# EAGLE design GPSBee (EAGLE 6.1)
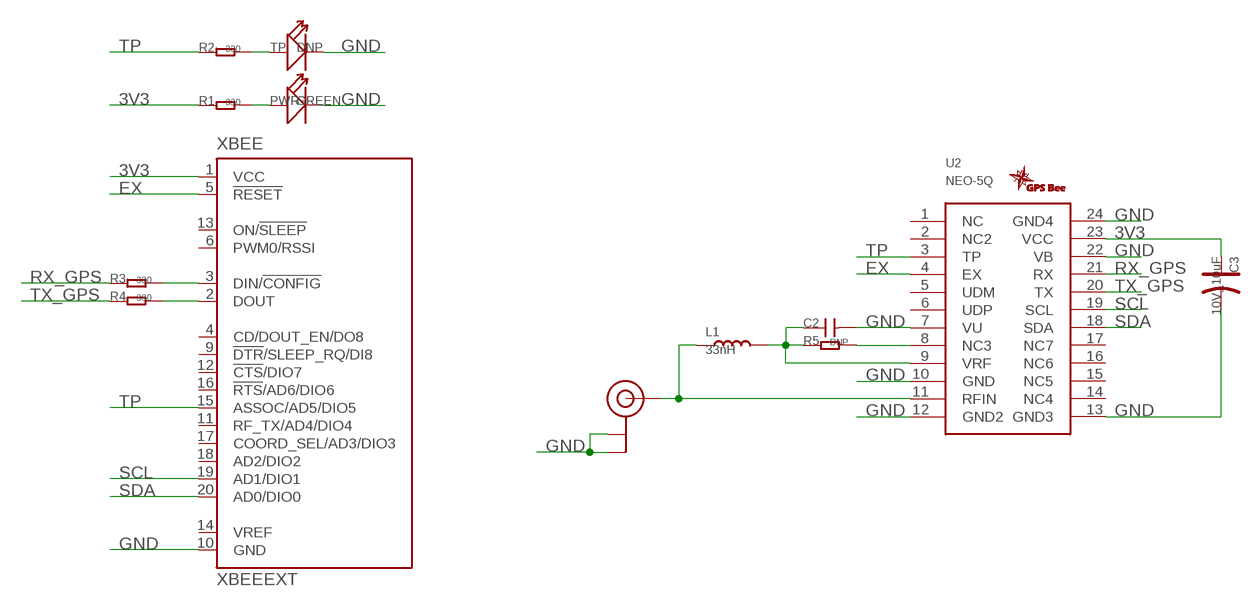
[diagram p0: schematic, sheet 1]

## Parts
C2  C-0603  [0603]
C3  10V_10uF  CAP-AVX-A  [AVX-A]
L1  33nH  L0603  [0603]
LOGO1  GPSLOGO_SLIK  [GPSLOGO]
PWR  GREEN  LED'0603'  [LED-0603]
R1  330  R-0603  [0603]
R2  330  R-0603  [0603]
R3  330  R-0603  [0603]
R4  330  R-0603  [0603]
R5  DNP  R-0603  [0603]
TP  DNP  LED'0603'  [LED-0603]
U2  NEO-5Q  [NEO-5Q]
U3  U.FL  [U.FL]
XBEE  XBEEEXT  [XBEE_PLUG]

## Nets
3V3: C3.+ R1.1 U2.23(VCC) XBEE.1(VCC)
EX: U2.4(EX) XBEE.5(!RESET)
GND: C2.2 C3.- PWR.- TP.- U2.7(VU) U2.10(GND) U2.12(GND2) U2.13(GND3) U2.22(VB) U2.24(GND4) U3.P$1(GND) U3.P$2(GND) XBEE.10(GND)
N$1: PWR.+ R1.2
N$2: L1.1 U2.11(RFIN) U3.P$3(SIGNAL)
N$3: C2.1 L1.2 R5.1 U2.9(VRF)
N$4: R3.2 XBEE.3(DIN/!CONFIG)
N$5: R2.2 TP.+
N$6: R4.2 XBEE.2(DOUT)
N$7: R5.2 U2.8(NC3)
RX_GPS: R3.1 U2.21(RX)
SCL: U2.19(SCL) XBEE.19(AD1/DIO1)
SDA: U2.18(SDA) XBEE.20(AD0/DIO0)
TP: R2.1 U2.3(TP) XBEE.15(ASSOC/AD5/DIO5)
TX_GPS: R4.1 U2.20(TX)
Unconnected: U2.1(NC) U2.2(NC2) U2.5(UDM) U2.6(UDP) U2.14(NC4) U2.15(NC5) U2.16(NC6) U2.17(NC7) XBEE.4(CD/DOUT_EN/DO8) XBEE.6(PWM0/RSSI) XBEE.9(!DTR!/SLEEP_RQ/DI8) XBEE.11(RF_TX/AD4/DIO4) XBEE.12(!CTS!/DIO7) XBEE.13(ON/!SLEEP) XBEE.14(VREF) XBEE.16(!RTS!/AD6/DIO6) XBEE.17(COORD_SEL/AD3/DIO3) XBEE.18(AD2/DIO2)

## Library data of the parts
C2 = Discrete:C*: Ceramic Capacitors
C3 = Discrete:CAP*: Electrolytic Capacitors,Tantalum Capacitors and Super Capacitors
L1 = Discrete:L*
LOGO1 = logo:GPSLOGO_SLIK
PWR TP = Discrete:LED*
R1-R5 = Discrete:R*
U2 = Seeed:NEO-5Q
U3 = SparkFun2:U.FL
XBEE = EXT_moudle:XBEE: XBee (TM) /XBee-PRO(TM) OEM RF Modules Source: MaxStream, Inc. xbee_productmanual.pdf

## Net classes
0 default: width 0.003 mm, drill 0.254 mm, clearance 0.152 mm

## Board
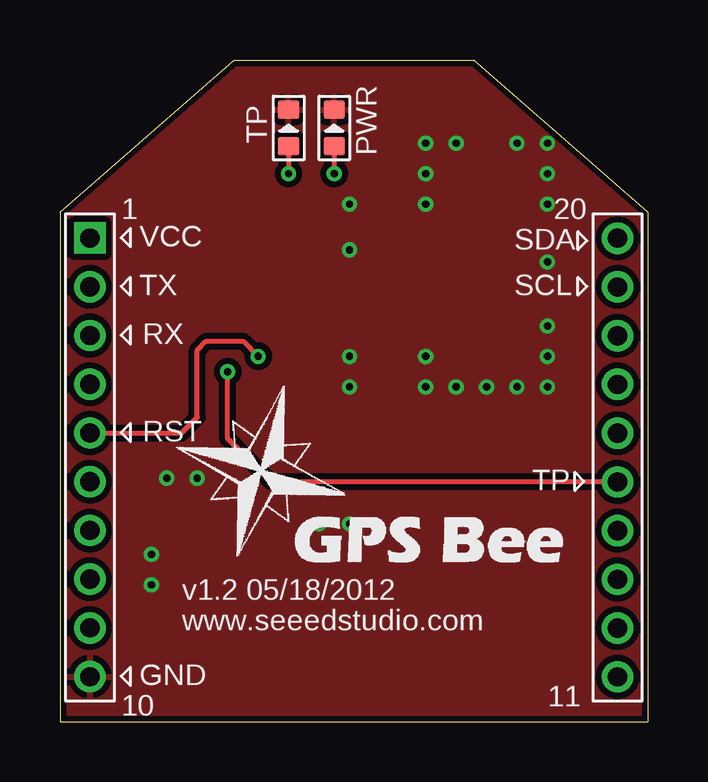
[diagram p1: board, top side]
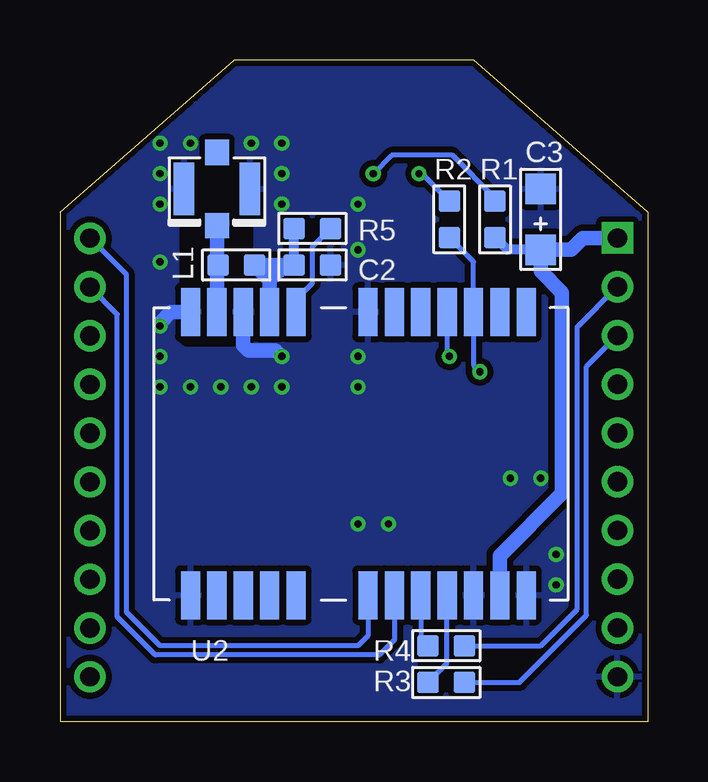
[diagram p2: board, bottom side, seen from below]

Size 24.5 x 27.6 mm. Coordinates in mm from the lower left corner, seen from the top.
Outline: 7.25,27.6 17.25,27.6 24.5,21.25 24.5,0 0,0 0,21.25 7.25,27.6
Copper layers (1*16): Top 0.035mm / dielectric 1.5mm / Bottom 0.035mm
Design rules: minimum track width 6mil, minimum drill 12mil, track to track 6mil, track to pad 6mil, pad to pad 6mil, via to via 6mil, smd to smd 0mil, copper to edge 10mil, drill to drill 10mil, minimum pad ring 10mil, minimum via ring 6mil, stop-mask expansion 2mil, vias tented up to drill 100mil, thermal gap 10mil
bRestrict: 4 lines

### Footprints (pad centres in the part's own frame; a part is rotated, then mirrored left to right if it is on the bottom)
0603 = smd 0.889 x 0.889: 1 -0.762,0; 2 0.762,0
AVX-A = smd 1.27 x 1.27: + -1.27,0; - 1.27,0
LED-0603 = smd 0.762 x 0.889: + -0.762,0; - 0.762,0
NEO-5Q = smd 2 x 0.8: 1 12,-14; 2 12,-12.9; 3 12,-11.8; 4 12,-10.7; 5 12,-9.6; 6 12,-8.5; 7 12,-7.4; 8 12,-4.4; 9 12,-3.3; 10 12,-2.2; 11 12,-1.1; 12 12,0; 13 0.2,0; 14 0.2,-1.1; 15 0.2,-2.2; 16 0.2,-3.3; 17 0.2,-4.4; 18 0.2,-7.4; 19 0.2,-8.5; 20 0.2,-9.6; 21 0.2,-10.7; 22 0.2,-11.8; 23 0.2,-12.9; 24 0.2,-14
U.FL = smd 2.2 x 0.85: P$1 0,1.375; P$2 0,-1.375 | smd 1.05 x 1: P$3 1.525,0; P$4 -1.525,0
XBEE_PLUG = drill 0.8 pad 1.27 square: 1 0,0.008 | drill 0.8 pad 1.27: 2 0,-2.024; 3 0,-4.056; 4 0,-6.088; 5 0,-8.12; 6 0,-10.152; 7 0,-12.184; 8 0,-14.216; 9 0,-16.248; 10 0,-18.28; 11 21.996,-18.288; 12 21.996,-16.256; 13 21.996,-14.224; 14 21.996,-12.192; 15 21.996,-10.16; 16 21.996,-8.128; 17 21.996,-6.096; 18 21.996,-4.064; 19 21.996,-2.032; 20 21.996,0

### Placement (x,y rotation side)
C2  13.98,19.05 0 bottom
C3  4.45,20.95 90 bottom
L1  17.15,19.05 0 bottom
LOGO1  4.45,5.71 0 top
PWR  11.44,24.77 90 top
R1  6.36,20.95 90 bottom
R2  8.26,20.95 90 bottom
R3  8.39,1.65 0 bottom
R4  8.39,3.17 0 bottom
R5  13.98,20.57 0 bottom
TP  9.53,24.77 90 top
U2  19.06,5.08 90 bottom
U3  17.96,22.23 270 bottom
XBEE  1.25,20.17 0 top

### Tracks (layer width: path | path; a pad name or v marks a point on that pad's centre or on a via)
3V3
  Bottom 0.406: C3.+ 5.85,19.68 R1.1
  Bottom 0.61: XBEE.1 2.69,20.18 3.18,19.68 C3.+ 4.45,18.8 3.56,17.91 3.56,9.53 6.16,6.93 U2.23
EX  (via drill 0.3 pad 0.64)
  Top 0.203: XBEE.5 5.07,12.05 5.72,12.7 5.72,15.49 6.1,15.88 7.63,15.88 v8.26,15.24
  Bottom 0.203: U2.4 8.36,15.34 v8.26,15.24
GND  (via drill 0.3 pad 0.64)
  Bottom 0.61: U2.12 19.88,17.08 20.33,16.64 v20.33,16.51 | U2.10 16.86,15.71 16.64,15.49 15.5,15.49 v15.25,15.24
  other vias: 15.25,21.59 15.25,22.86 15.25,24.13 16.52,24.13 20.33,24.13 20.33,22.86 20.33,21.59 20.33,15.24 19.06,13.97 17.79,13.97 16.52,13.97 15.25,13.97 20.33,19.18 19.06,24.13 20.33,13.97 3.82,6.99 5.72,10.16 3.82,5.71 4.45,10.16 10.8,8.26 12.07,15.24 12.07,13.97 12.07,19.68 12.07,21.59 12.07,8.26
  pour Bottom (isolate 0.254): 0.01,27.94 24.77,27.94 24.77,0 0.01,0
  pour Top (isolate 0.254): 0.01,27.94 24.77,27.94 24.77,0 0.01,0
N$1  (via drill 0.3 pad 0.64)
  Top 0.203: PWR.+ v11.44,22.86
  Bottom 0.203: R1.2 6.36,21.84 8.14,23.62 10.68,23.62 v11.44,22.86
N$2
  Bottom 0.61: U3.P$3 U2.11 17.96,19.01 L1.1
N$3
  Bottom 0.406: C2.1 R5.1
  Bottom 0.61: U2.9 15.76,18.42 | 15.76,18.42 L1.2 15.12,19.05 | C2.1 14.87,19.05 15.12,19.05 | 15.12,19.05 15.76,18.42
N$4
  Bottom 0.203: XBEE.3 2.55,14.82 2.55,4.45 5.34,1.65 R3.2
N$5  (via drill 0.3 pad 0.64)
  Top 0.203: TP.+ v9.53,22.86
  Bottom 0.203: v9.53,22.86 9.41,22.86 R2.2
N$6
  Bottom 0.203: R4.2 4.45,3.17 2.93,4.7 2.93,16.47 XBEE.2
N$7
  Bottom 0.203: U2.8 14.66,17.61 13.98,18.29 13.98,19.81 R5.2
RX_GPS
  Bottom 0.203: U2.21 8.36,4.48 8.39,4.45 8.39,2.41 R3.1
SCL
  Bottom 0.203: U2.19 10.56,3.42 11.18,2.79 20.53,2.79 22.11,4.37 22.11,16.99 XBEE.19
SDA
  Bottom 0.203: U2.18 11.66,3.59 12.07,3.17 20.33,3.17 21.72,4.57 21.72,18.64 XBEE.20
TP  (via drill 0.3 pad 0.64)
  Top 0.203: XBEE.15 8.8,10.01 6.99,11.81 v6.99,14.61
  Bottom 0.203: R2.1 7.26,19.19 U2.3 7.26,14.87 v6.99,14.61
TX_GPS
  Bottom 0.203: U2.20 9.46,3.48 R4.1

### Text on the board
tPlace: 1 | 20 | VCC | SDA | TX | SCL | RX | RST | TP | v1.2 05/18/2012 | www.seeedstudio.com | GND | 11 | 10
